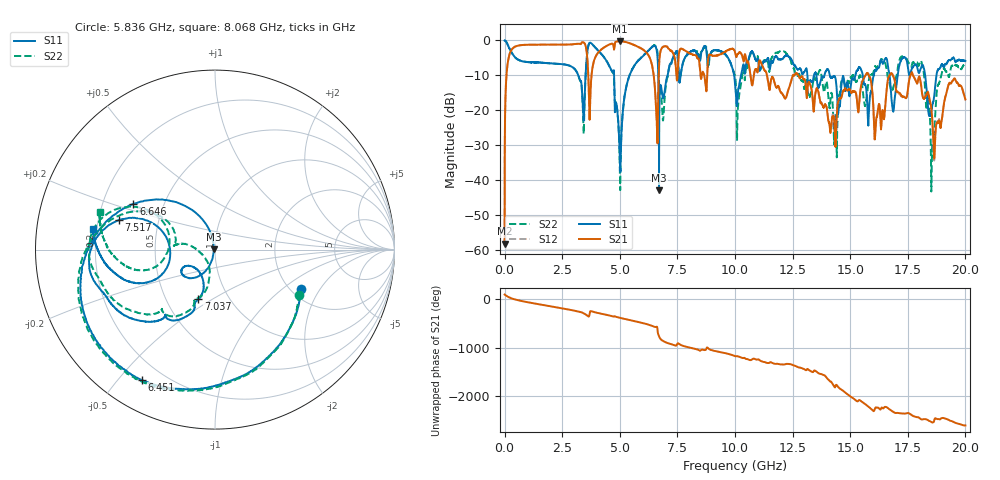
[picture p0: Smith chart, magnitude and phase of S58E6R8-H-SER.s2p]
!{S58E6R8}
!Johanson Technology Inc.
!www.johansontechnology.com
!Test Board Conditions:
!Substrate Type  RO4350B
!Substrate Thickness  60 mil
!Substrate Dk  3.66
!TL Type: GCPW
!TL Trace Width  115 mil
!TL Gap  52 mil
!Electrode orientation  Horizontal
!DUT TOPOLOGY	SERIES
!Mounting Pad LxW  55x428 mil
! Created Tue Apr 13 22:43:00 2021
# hz S ma R 50
! 2 Port Network Data from SP1.SP block
! freq  magS11  angS11  magS21  angS21  magS12  angS12  magS22  angS22
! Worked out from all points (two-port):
!   20001 points, 300 kHz to 20 GHz, reference 50 ohm
!   highest |S21| = -0.23 dB at 4.99 GHz (marker M1); lowest = -58.1 dB at 300 kHz (marker M2)
!   |S21| within 3 dB of the highest: 251.9 MHz to 3.563 GHz (3.311 GHz wide, 174 % of centre); 4.093 GHz to 6.121 GHz (2.028 GHz wide, 39.7 % of centre)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
!   lowest |S11| = -42.8 dB at 6.703 GHz (marker M3), VSWR 1.01, Z = 49.3 + j0.146 ohm
!   |S11| at or under -10 dB: 4.753 GHz to 5.422 GHz (668.7 MHz wide, 13.1 % of centre); 14.11 GHz to 15.22 GHz (1.113 GHz wide, 7.59 % of centre); 18.25 GHz to 18.74 GHz (487.1 MHz wide, 2.63 % of centre)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
!   |S22| runs from -43.2 to 0.0 dB; largest |S21 - S12| = 0.011
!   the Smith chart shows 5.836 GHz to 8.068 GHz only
!   S11 on the Smith chart (normalised r, x): 5.836 GHz: 2.26, -1.37; 6.451 GHz: 0.12, -0.58; 6.646 GHz: 0.33, +0.23; 7.037 GHz: 0.72, -0.44; 7.517 GHz: 0.29, +0.14; 8.068 GHz: 0.18, +0.08
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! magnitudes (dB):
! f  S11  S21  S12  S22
! 300 kHz  0.0  -58.1  -58.8  0.0
! 111.3 MHz  -0.9  -7.7  -7.7  -0.9
! 301.3 MHz  -3.4  -2.6  -2.6  -3.4
! 3.334 GHz  -12.2  -0.7  -0.7  -12.4
! 4.273 GHz  -4.4  -2.2  -2.2  -4.4
! 4.99 GHz  -31.3  -0.2  -0.2  -32.6
! 5.836 GHz  -5.6  -1.9  -1.9  -5.5
! 6.451 GHz  -1.6  -8.9  -8.9  -1.6
! 6.646 GHz  -5.7  -26.3  -25.8  -3.8
! 6.667 GHz  -9.1  -16.2  -16.1  -5.9
! 6.703 GHz  -42.8  -7.3  -7.3  -12.2
! 7.037 GHz  -10.7  -1.7  -1.7  -11.2
! 7.517 GHz  -5.0  -8.2  -8.2  -5.0
! 8.068 GHz  -3.2  -3.8  -3.7  -3.4
! 10 GHz  -12.2  -3.3  -3.4  -10.3
! 13.33 GHz  -11.9  -14.5  -14.3  -14.0
! 14.36 GHz  -10.7  -30.0  -29.8  -21.5
! 16.67 GHz  -8.5  -10.5  -10.5  -11.2
! 18.09 GHz  -7.5  -13.5  -13.4  -6.1
! 18.57 GHz  -18.3  -23.5  -23.8  -29.6
! 18.99 GHz  -6.8  -21.9  -22.0  -8.9
! 20 GHz  -5.9  -16.8  -16.9  -6.2
